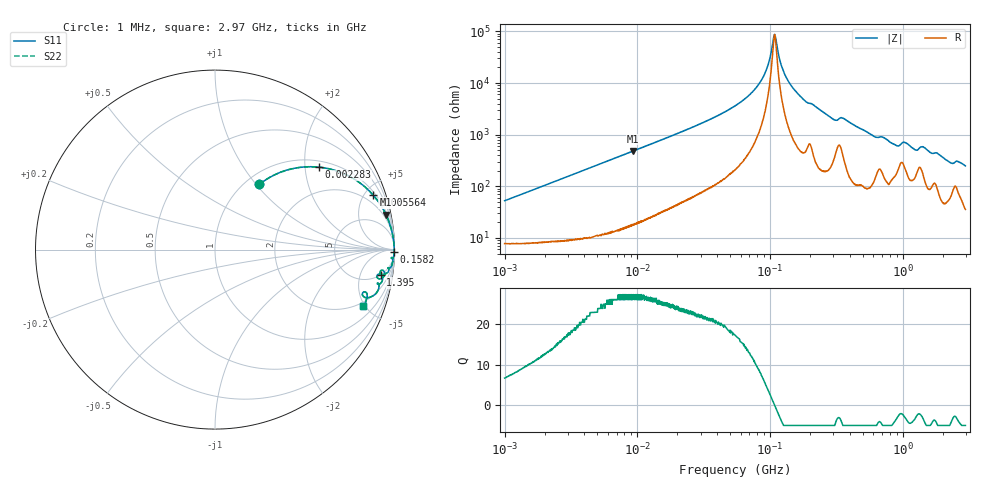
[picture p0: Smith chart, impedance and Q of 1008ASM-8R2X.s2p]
!s-Parameter Generated by FASTRON Sdn. Bhd.
!FASTRON P/N : 1008ASM-8R2X
!Keysight Technologies: E4991B_MY54100416_A.01.15
!Date: Tue Nov 21 10:21:14 2023
!Version  :Rev00  Wed Nov 22 15:10:30 2023
!Data & Calibration Information:
!Freq  S11  S21  S12  S22
!PortZ  Port1:50+j0  Port2:50+j0
!When reading reference impedance value at option line is always used.
! Remarks : This data is being provided solely for informational purposes.
# Hz S dB R 50
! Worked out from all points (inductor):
!   1599 points, 1 MHz to 2.97 GHz, reference 50 ohm
!   read as one part in series: L = 8.27 uH near 1.036 MHz
!   highest Q = 27.3 at 9.316 MHz (marker M1), where L = 8.22 uH
!   self-resonance near 108.2 MHz
!   S11 on the Smith chart (normalised r, x): 1 MHz: 1.16, +1.04; 2.283 MHz: 1.17, +2.37; 5.564 MHz: 1.23, +5.75; 158.2 MHz: open; 1.395 GHz: 5, -11; 2.97 GHz: 1.71, -4.90
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1000000  -7.14 55.7  -1.56 -25.8  -1.56 -25.8  -7.14 55.7
2283380  -2.63 38.4  -4.12 -47.5  -4.12 -47.5  -2.63 38.4
3804036  -1.16 26.3  -7.06 -60.9  -7.06 -60.9  -1.16 26.3
5564266  -0.60 18.9  -9.80 -68.8  -9.80 -68.8  -0.60 18.9
9316388  -0.25 11.6  -13.90 -76.3  -13.90 -76.3  -0.25 11.6
1.439846e7  -0.12 7.6  -17.60 -80.2  -17.60 -80.2  -0.12 7.6
5.477226e7  -0.02 1.6  -31.20 -85.1  -31.20 -85.1  -0.02 1.6
7.176513e7  -0.01 0.9  -36.00 -84.4  -36.00 -84.4  -0.01 0.9
8.636184e7  -0.01 0.5  -41.20 -81.7  -41.20 -81.7  -0.01 0.5
9.641227e7  -0.01 0.3  -46.80 -75.2  -46.80 -75.2  -0.01 0.3
1.081723e8  -0.01 0.0  -58.80 -3.8  -58.80 -3.8  -0.01 0.0
1.275944e8  -0.01 -0.4  -44.00 78.9  -44.00 78.9  -0.01 -0.4
1.582265e8  -0.01 -0.9  -36.50 83.9  -36.50 83.9  -0.01 -0.9
2.073156e8  -0.03 -1.4  -31.90 81.1  -31.90 81.1  -0.03 -1.4
3.032461e8  -0.09 -2.9  -25.90 77.4  -25.90 77.4  -0.09 -2.9
3.541315e8  -0.09 -2.7  -26.50 76.4  -26.50 76.4  -0.09 -2.7
7.846996e8  -0.24 -7.4  -17.80 74.4  -17.80 74.4  -0.24 -7.4
9.072485e8  -0.52 -8.5  -16.20 63.8  -16.20 63.8  -0.52 -8.5
1.033307e9  -0.46 -7.3  -17.50 63.7  -17.50 63.7  -0.46 -7.3
1.249715e9  -0.65 -10.1  -14.70 62.1  -14.70 62.1  -0.65 -10.1
1.395152e9  -0.59 -8.6  -15.90 61.4  -15.90 61.4  -0.59 -8.6
2.970126e9  -1.07 -20.7  -8.95 61.0  -8.95 61.0  -1.07 -20.7
